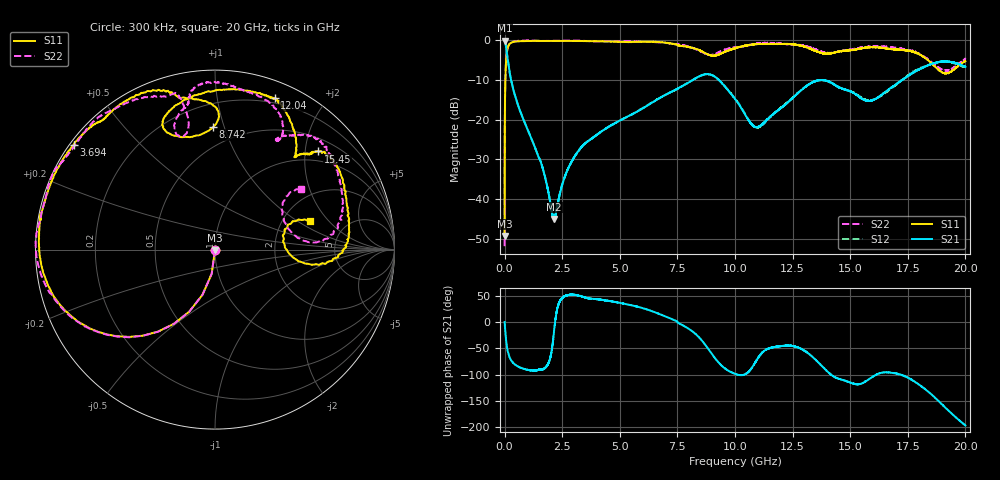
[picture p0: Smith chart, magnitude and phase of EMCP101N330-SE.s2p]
!EMCP101N330
!Johanson Technology Inc.
!www.johansontechnology.com
!Test Board Conditions:
!Substrate Type  RO4350B
!Substrate Thickness  10 mil
!Substrate Dk  3.66
!TL Type: GCPW
!TL Trace Width  20 mil
!TL Gap  10 mil
!PART MODE SINGLE ENDED (AKA BYPASS)
!DUT TOPOLOGY	SERIES-SHUNT
# MHz S  dB  R 50
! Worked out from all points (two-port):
!   20001 points, 300 kHz to 20 GHz, reference 50 ohm
!   highest |S21| = -0.01 dB at 300 kHz (marker M1); lowest = -45.1 dB at 2.15 GHz (marker M2)
!   |S21| within 3 dB of the highest: start of sweep to 95.22 MHz
!   lowest |S11| = -49.3 dB at 300 kHz (marker M3), VSWR 1.01, Z = 50 - j0.341 ohm
!   |S11| at or under -10 dB: start of sweep to 32.45 MHz
!   |S22| runs from -51.9 to 0.0 dB; largest |S21 - S12| = 0.017
!   S11 on the Smith chart (normalised r, x): 300 kHz: 1.00, -0.01; 3.694 GHz: 0.01, +0.33; 8.742 GHz: 0.36, +0.92; 12.04 GHz: 0.16, +1.46; 15.45 GHz: 0.77, +2.27; 20 GHz: 2.78, +1.30
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0.3  -49.30 -95.8  -0.01 0.0  -0.00 -0.2  -51.89 -85.9
103.298  -2.79 -138.2  -3.38 -47.7  -3.35 -47.6  -2.79 -138.0
190.297  -1.06 -155.4  -7.03 -64.3  -7.00 -64.3  -1.07 -154.9
377.294  -0.37 -170.1  -12.34 -78.0  -12.31 -78.2  -0.30 -168.7
830.288  -0.15 177.2  -20.11 -89.0  -20.15 -89.0  -0.01 179.4
1616.276  -0.13 169.7  -31.50 -90.7  -31.46 -90.4  -0.10 166.6
2150.268  -0.12 165.7  -45.05 -15.7  -44.88 -16.5  -0.09 160.7
2679.26  -0.12 159.5  -33.39 50.5  -33.38 50.2  -0.03 156.5
3334.25  -0.14 149.0  -26.91 49.0  -26.91 49.0  -0.07 152.2
3694.245  -0.17 143.4  -25.08 44.7  -25.10 44.9  -0.16 149.9
6667.2  -0.36 113.3  -14.76 16.2  -14.70 15.8  -0.47 118.6
7600.186  -1.29 101.2  -11.85 -3.1  -11.85 -2.9  -1.00 103.6
8742.169  -3.30 90.9  -8.49 -45.2  -8.53 -45.3  -3.41 103.2
10000.15  -1.98 110.2  -14.74 -98.6  -14.59 -98.1  -1.75 101.3
10921.14  -0.92 83.5  -21.84 -73.9  -21.93 -75.1  -0.83 97.2
12038.12  -0.86 68.5  -16.86 -45.6  -16.77 -44.9  -0.84 81.8
13334.1  -2.25 54.7  -10.65 -65.2  -10.64 -65.5  -1.90 62.1
15449.07  -2.02 43.6  -14.47 -117.8  -14.28 -117.5  -1.81 51.8
16667.05  -2.10 21.9  -12.35 -96.0  -12.61 -95.7  -1.65 37.8
18393.02  -5.08 -8.6  -6.23 -132.6  -6.16 -133.5  -4.82 4.3
19170.01  -8.28 7.8  -5.28 -164.5  -5.34 -165.3  -7.61 22.3
20000  -5.17 17.1  -6.66 163.2  -6.88 164.3  -4.53 35.3
